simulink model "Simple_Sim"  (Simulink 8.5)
settings: Solver=ode45  StartTime=0.0  StopTime=20000  MaxStep=1  RelTol=1e-3
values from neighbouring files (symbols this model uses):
  Kpqr = lqr(sys,Q0,R0)    [des.m]
  wo = 0.0011    [start.m]    (also in start1.m; start2.m; start3.m)
undefined symbols (not defined in the file or in its folder): A0, B0, C0, D0

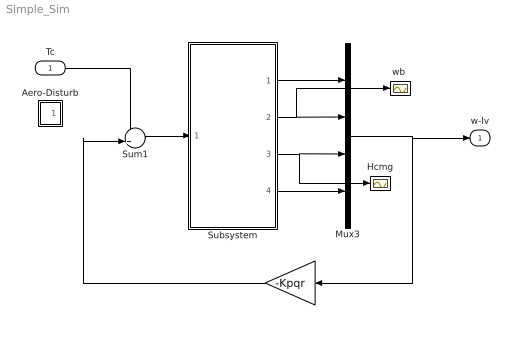
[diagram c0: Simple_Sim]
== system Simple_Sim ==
  Tc : Inport  PortDimensions=3
  " " : Gain  Gain=-Kpqr  Multiplication=Matrix(K*u)
  Aero-Disturb : Subsystem
  Hcmg : Scope
  Mux3 : Mux  Inputs=[3, 3, 3, 3]
  Subsystem : Subsystem
  Sum1 : Sum  Inputs=++|
  "wb " : Scope
  w-lv : Outport
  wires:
  Subsystem/4(H-Integr) -> Mux3/4
  Subsystem/3(H-cmg) -> Hcmg/1, Mux3/3
  Mux3/1 -> " "/1, w-lv/1
  Sum1/1 -> Subsystem/1(Tc)
  " "/1 -> Sum1/2
  Subsystem/2(wl) -> "wb "/1, Mux3/2
  Subsystem/1(atti-lv) -> Mux3/1
  Tc/1 -> Sum1/1

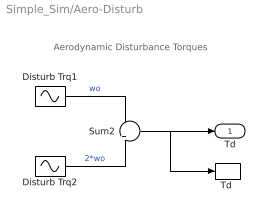
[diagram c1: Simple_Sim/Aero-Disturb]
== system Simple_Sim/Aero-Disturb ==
  note: Aerodynamic Disturbance Torques
  Disturb Trq1 : Sin  Amplitude=[1, 3, 1]  Bias="[1  8  1]"  Frequency=[wo, wo, wo]  SampleTime=0
  Disturb Trq2 : Sin  Amplitude=[1, 1, 1]*0.5  Frequency=[wo, wo, wo]*2  SampleTime=0
  Sum2 : Sum  Inputs=+|+
  "Td " : ToWorkspace  VariableName=Td  SampleTime=-1
  Td : Outport
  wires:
  Disturb Trq2/1 -> Sum2/2  "2*wo"
  Sum2/1 -> "Td "/1, Td/1
  Disturb Trq1/1 -> Sum2/1  "wo"

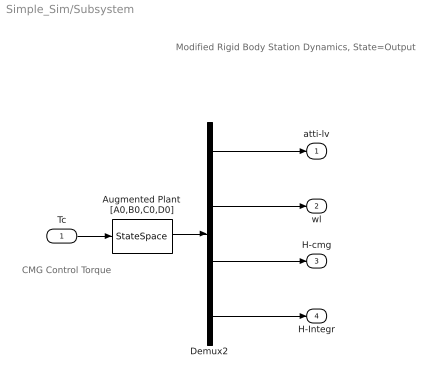
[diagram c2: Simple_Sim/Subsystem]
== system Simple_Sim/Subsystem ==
  note: Modified Rigid Body Station Dynamics, State=Output
  note: CMG Control Torque
  Tc : Inport  PortDimensions=3
  Augmented Plant [A0,B0,C0,D0] : StateSpace  A=A0  B=B0  C=C0  D=D0  X0=0
  Demux2 : Demux  Outputs=[3, 3, 3, 3]
  atti-lv : Outport
  wl : Outport  Port=2
  H-cmg : Outport  Port=3
  H-Integr : Outport  Port=4
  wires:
  Demux2/2 -> wl/1
  Tc/1 -> Augmented Plant [A0,B0,C0,D0]/1
  Demux2/1 -> atti-lv/1
  Demux2/3 -> H-cmg/1
  Demux2/4 -> H-Integr/1
  Augmented Plant [A0,B0,C0,D0]/1 -> Demux2/1
